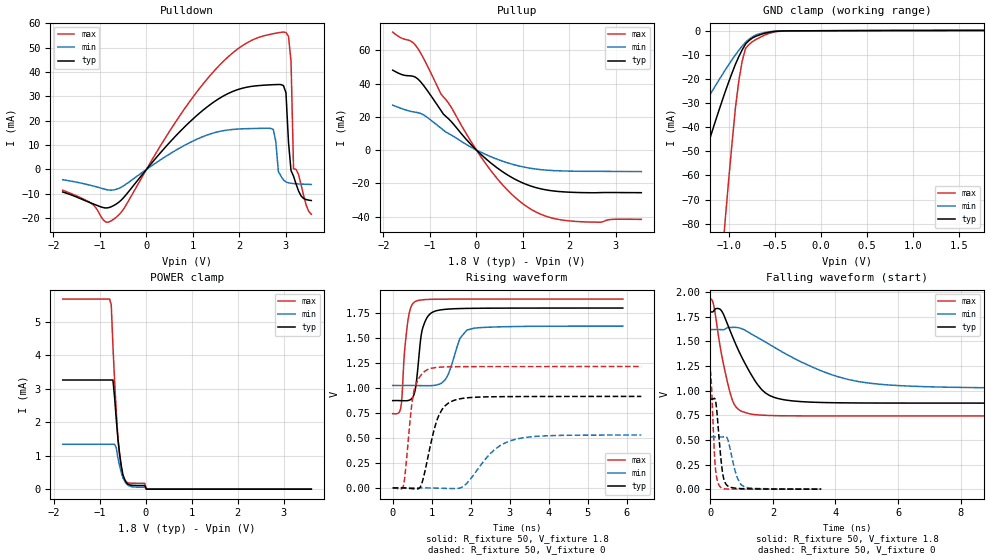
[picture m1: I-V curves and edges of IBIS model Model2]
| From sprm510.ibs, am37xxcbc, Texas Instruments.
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| Model based on original model for BQ18OMAPJTAGFBPBNOPM_SSBHV
|   Sub model AGFBPBNOPM_VJTAG_PD1_1P8
[model]   Model2
|[Input Load]   PD
|[Output Drive]
|Voltage   1.8V
|Mode   I/O
Model_type   I/O
Polarity   Non-Inverting
Enable   Active-Low
Vinl =  0.63
Vinh =  1.17
Cref =  15pF
Rref =  100.0000M
Vref =  0V
Vmeas =  0.9
C_comp   2.132351p   1.924211p   2.13513p
[Model Spec]
Vinl   0.63   0.567   0.6615
Vinh   1.17   1.053   1.2285
[Temperature Range]   25   125   -40
[Voltage Range]   1.8   1.62   1.89
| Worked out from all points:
|   slope of the pulldown table from 0 to 0.27 V, typ, clamps not added: 43.9 ohm
|   slope of the pullup table from 0 to 0.27 V, typ, clamps not added: 39.4 ohm
|   GND clamp passes 1 mA (typ) near -0.61 V on its own axis
|   POWER clamp passes 1 mA (typ) near -0.56 V on its own axis
|   rising waveform, R_fixture 50, V_fixture 1.8: 20-80 % time 175ps typ, 301ps min, 139ps max; typ from 0.872 V to 1.8 V
|   rising waveform, R_fixture 50, V_fixture 0: 20-80 % time 356ps typ, 725ps min, 201ps max; typ from 0 V to 0.914 V
|   falling waveform, R_fixture 50, V_fixture 1.8: 20-80 % time 893ps typ, 2.32ns min, 433ps max; typ from 1.8 V to 0.873 V
|   falling waveform, R_fixture 50, V_fixture 0: 20-80 % time 160ps typ, 253ps min, 106ps max; typ from 0.915 V to 0 V
[POWER_clamp]
-1.8V     3.257mA    1.34mA     5.672mA
-781.8mV  3.257mA    1.34mA     5.672mA
-745.5mV  3.257mA    1.34mA     5.502mA
-709.1mV  3.257mA    1.34mA     4.272mA
-636.4mV  2.077mA    1.231mA    2.311mA
-600mV    1.485mA    926.4uA    1.517mA
-527.3mV  696.2uA    496.1uA    625.9uA
-490.9mV  425.4uA    335.1uA    371.7uA
-418.2mV  198.1uA    164.6uA    216.5uA
-18.18mV  109.6uA    59.03uA    175uA
18.18mV   0A         0A         0A
3.6V      0A         0A         0A
[Pulldown]
-1.8V     -9.247mA   -4.208mA   -8.543mA
-709.1mV  -14.86mA   -8.413mA   -20.46mA
927.3mV   19.42mA    10.96mA    27.78mA
1.964V    32.76mA    16.57mA    49.44mA
2.727V    34.78mA    16.43mA    55.71mA
2.836V    34.85mA    -785uA     56.1mA
2.945V    34.44mA    -4.282mA   56.36mA
3V        31.5mA     -5.132mA   56.19mA
3.055V    11.24mA    -5.498mA   54.62mA
3.109V    -463.9uA   -5.674mA   44.42mA
3.164V    -2.788mA   -5.786mA   273.8uA
3.545V    -12.75mA   -6.152mA   -18.39mA
[Pullup]
-1.8V     48.03mA    26.96mA    70.92mA
-1.309V   43.76mA    22.71mA    63.01mA
-1.145V   39.16mA    21.26mA    55.56mA
-763.6mV  23.82mA    13.18mA    33.74mA
-545.5mV  17.24mA    9.103mA    25.87mA
54.55mV   -1.471mA   -757.9uA   -2.315mA
545.5mV   -12.73mA   -6.543mA   -20.39mA
981.8mV   -19.62mA   -10.01mA   -31.96mA
1.418V    -23.55mA   -11.89mA   -39.01mA
1.855V    -25.13mA   -12.59mA   -42.14mA
2.673V    -25.59mA   -12.83mA   -43.4mA
3.545V    -25.66mA   -12.97mA   -41.71mA
[GND_clamp]
-1.8V     -118.7mA   -65.68mA   -455.2mA
-1.509V   -82.26mA   -46.44mA   -309.2mA
-1.473V   -77.72mA   -44.04mA   -290.9mA
-1.073V   -29.19mA   -18.4mA    -94.44mA
-1.036V   -25.09mA   -16.2mA    -77.62mA
-927.3mV  -13.89mA   -9.972mA   -31.97mA
-890.9mV  -10.73mA   -8.113mA   -20.85mA
-854.5mV  -7.95mA    -6.383mA   -12.63mA
-818.2mV  -5.532mA   -4.782mA   -7.33mA
-745.5mV  -3.063mA   -2.571mA   -4.597mA
-418.2mV  -94.1uA    -65.98uA   -158.2uA
1.764V    109.6uA    59.69uA    174.8uA
[Ramp]
dV/dt_f  0.5755053/0.9114897n  0.3701856/2.38504n   0.7114036/0.4330493n
dV/dt_r  0.5550131/0.3572719n  0.3218817/0.7339067n  0.7353063/0.2014578n
R_load = 50
[Rising Waveform]
R_fixture = 50
V_fixture = 1.8
V_fixture_min = 1.62
V_fixture_max = 1.89
0s        872.4mV    1.024V     742.3mV
207ps     872.1mV    1.023V     800.5mV
303ps     871mV      1.024V     1.364V
381ps     872.2mV    1.024V     1.646V
579ps     985.3mV    1.023V     1.862V
756ps     1.58V      1.022V     1.88V
1.062ns   1.763V     1.024V     1.885V
1.392ns   1.786V     1.111V     1.886V
1.899ns   1.794V     1.577V     1.887V
5.895ns   1.797V     1.617V     1.887V
[Rising Waveform]
R_fixture = 50
V_fixture = 0
V_fixture_min = 0
V_fixture_max = 0
0s        -415.3uV   95.87uV    101.4uV
270ps     -15.58uV   -462.5uV   14.99mV
474ps     -6.526mV   103.7uV    784.5mV
543ps     -9.191mV   102.8uV    966.1mV
735ps     31.97mV    84.19uV    1.131V
897ps     298.1mV    -138uV     1.183V
1.185ns   727.3mV    -2.954mV   1.206V
1.653ns   884.3mV    -6.297mV   1.211V
3.051ns   912.5mV    475.7mV    1.212V
6.369ns   914.2mV    528.1mV    1.213V
[Falling Waveform]
R_fixture = 50
V_fixture = 1.8
V_fixture_min = 1.62
V_fixture_max = 1.89
0s        1.798V     1.618V     1.928V
105ps     1.804V     1.619V     1.873V
342ps     1.815V     1.618V     1.397V
678ps     1.572V     1.64V      928.6mV
852ps     1.442V     1.639V     822.8mV
1.203ns   1.22V      1.594V     768.1mV
1.638ns   1.011V     1.515V     750.5mV
2.145ns   920.7mV    1.42V      745.1mV
4.734ns   874.1mV    1.091V     742.7mV
12.35ns   872.7mV    1.025V     742.7mV
[Falling Waveform]
R_fixture = 50
V_fixture = 0
V_fixture_min = 0
V_fixture_max = 0
0s        914.7mV    529.6mV    1.205V
39ps      914.1mV    529.6mV    1.048V
120ps     918.9mV    530.1mV    443.8mV
165ps     900.9mV    530.2mV    210.5mV
324ps     360.2mV    529.3mV    20.82mV
405ps     143.1mV    529.8mV    6.091mV
504ps     50.07mV    532.2mV    2.164mV
870ps     7.977mV    110.2mV    546.2uV
1.092ns   4.286mV    22.45mV    315.5uV
3.543ns   298uV      1.623mV    3.389uV
